FUNCTION_BLOCK FB_TEST
VAR_INPUT
	{attribute 'OPC.UA.DA' := '1'}
	nInput1		: INT; (*~ (OPC:1:available) *)
	nInput2		: INT;
END_VAR
VAR_OUTPUT
	{attribute 'OPC.UA.DA' := '1'}
	nOutput1 	: INT;
	nOutput2 	: INT;
END_VAR
VAR
	{attribute 'OPC.UA.DA' := '1'}
	nVariable 	: INT;
END_VAR

nVariable := nInput1 + nInput2;
nOutput1 := nVariable + nInput1;
nOutput2 := nVariable + nInput2;

END_FUNCTION_BLOCK
